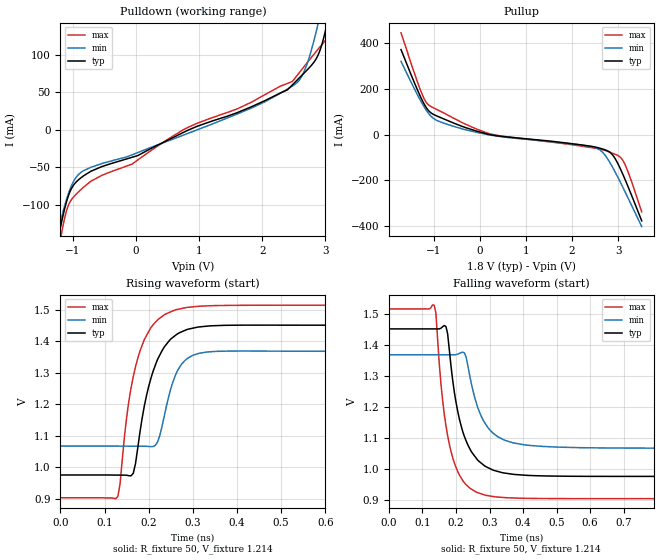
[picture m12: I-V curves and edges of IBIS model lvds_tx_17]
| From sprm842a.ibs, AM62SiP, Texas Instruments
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|   MODEL lvds_tx_17
[Model] lvds_tx_17
Model_type Output
C_comp 1.664p 1.756p 1.468p
Vmeas = 1.2
Vref = 1.2V
Rref = 50
Cref = 0.5pF
[Model Spec]
[Temperature Range]  40 150 -40
[Voltage Range] 1.8 1.62 1.98
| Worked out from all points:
|   slope of the pulldown table from 0 to 0.27 V, typ, clamps not added: 23.2 ohm
|   slope of the pullup table from 0 to 0.27 V, typ, clamps not added: 20.1 ohm
|   rising waveform, R_fixture 50, V_fixture 1.214: 20-80 % time 49ps typ, 36ps min, 46.5ps max; typ from 0.975 V to 1.45 V
|   falling waveform, R_fixture 50, V_fixture 1.214: 20-80 % time 55.6ps typ, 59.7ps min, 46.3ps max; typ from 1.45 V to 0.975 V
[Pulldown]
-1.71V    -377.9mA   -327mA     -450.4mA
-1.245V   -149.2mA   -138.6mA   -169.8mA
-1.182V   -123mA     -116.6mA   -138mA
-1.034V   -79.84mA   -76.3mA    -94.23mA
-828.4mV  -61.16mA   -54.3mA    -76.13mA
2.043V    38.71mA    37.15mA    46.68mA
2.587V    68.85mA    65.58mA    75.71mA
2.729V    80.97mA    91.83mA    90.91mA
2.872V    96.83mA    136.1mA    105.7mA
3.03V     141.9mA    196.2mA    121.7mA
3.125V    182.3mA    234.7mA    136.4mA
3.511V    372.1mA    396.2mA    335.4mA
[Pullup]
-1.711V   372.1mA    320.5mA    445.6mA
-1.299V   170.5mA    153.1mA    200mA
-1.188V   126.4mA    114.5mA    149.1mA
-1.098V   101.7mA    89.06mA    127.6mA
-750mV    65.7mA     47.68mA    90.96mA
214.2mV   0A         -1.715mA   3.373mA
2.565V    -57.7mA    -62.75mA   -62.4mA
2.702V    -66.01mA   -87.26mA   -68.95mA
2.855V    -83.97mA   -135mA     -79.92mA
3.088V    -168.1mA   -225.5mA   -109.2mA
3.225V    -233.7mA   -282.6mA   -169.6mA
3.51V     -377.9mA   -403mA     -338.4mA
[Ramp]
dV/dt_r .286/49.205p .181/35.971p .369/46.704p
dV/dt_f .286/55.6p .181/59.485p .369/45.953p
[Rising Waveform]
R_fixture = 50
V_fixture = 1.214
V_fixture_min = 1.218
V_fixture_max = 1.21
0s        975.4mV    1.067V     902.9mV
130ps     975mV      1.067V     906.8mV
150ps     974.6mV    1.067V     1.159V
165ps     980.7mV    1.067V     1.288V
180ps     1.11V      1.067V     1.369V
200ps     1.257V     1.066V     1.432V
220ps     1.343V     1.08V      1.468V
255ps     1.413V     1.272V     1.497V
285ps     1.437V     1.343V     1.508V
2.555ns   1.452V     1.369V     1.516V
[Falling Waveform]
R_fixture = 50
V_fixture = 1.214
V_fixture_min = 1.218
V_fixture_max = 1.21
0s        1.453V     1.369V     1.517V
135ps     1.453V     1.369V     1.53V
170ps     1.46V      1.369V     1.139V
190ps     1.287V     1.369V     1.036V
225ps     1.104V     1.375V     954.1mV
260ps     1.034V     1.215V     924.3mV
290ps     1.006V     1.142V     913.4mV
350ps     984.9mV    1.09V      905.9mV
505ps     975.8mV    1.07V      903mV
2.555ns   975.3mV    1.067V     902.7mV
